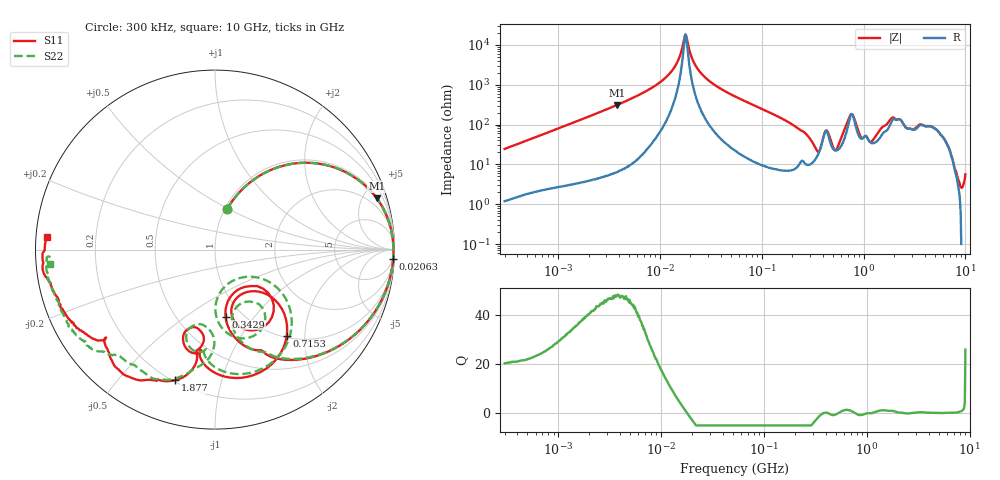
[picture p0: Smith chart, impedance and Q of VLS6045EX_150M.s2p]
! S-Parameter Data Generated by TDK Corporation
! Copyright(C) 2019 TDK Corporation.
! All Rights Reserved.
! TDK P/N: VLS6045EX-150M (Inductor)
! Property: L=15uH at 100kHz
! Size(LxWxT): 6x6x4.5mm
! Model Type: s2p (Touchstone File Format Version 1.0)
! Frequency: DC=Yes Start=0.3MHz Stop=10000MHz 802points Log-sweep
! Model Generated on May 10, 2019
! Port Assignments:
!  1 ---@@@--- 2
! Applicable Conditions:
!  Temperature = 25 degC
!  DC Bias Current = 0 A
!  Small Signal Operation
! Terms and conditions regarding TDK Simulation Models
! (1)This simulation model is being provided solely for informational purposes. Please refer to the specifications of the products in terms of detailed characteristics of such products.
! (2)In no event shall TDK Corporation of any of its subsidiaries be liable for any loss or damage arising, directly or indirectly,
!  From any information contained in this simulation model, including, but not limited to loss or damages arising from any inaccuracies, omissions or errors in connection with such information.
! (3)Any and all copyrights on this simulation model are owned by TDK Corporation.
!  Duplication or redistribution of this simulation model without prior written permission from TDK Corporation is prohibited.
! (4)This simulation model is subject to any modification or change without any prior notice.
! (5)Neither TDK Corporation nor any of its subsidiaries shall make any warranty, express or implied,
!  Including but not limited to the correctness, implied warranties of merchantability and fitness for a particular purpose with respect to this simulation models.
! (6)The use of this simulation model shall be deemed to have consented to the terms and conditions hereof.
# Hz S MA R 50
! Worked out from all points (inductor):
!   801 points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, 300 kHz to 10 GHz, reference 50 ohm
!   read as one part in series: L = 12.9 uH near 318.3 kHz
!   highest Q = 48 at 3.777 MHz (marker M1), where L = 12.9 uH
!   self-resonance near 17.86 MHz
!   S11 on the Smith chart (normalised r, x): 300 kHz: 1.03, +0.49; 20.63 MHz: 4, -38; 342.9 MHz: 0.84, -0.73; 715.3 MHz: 1.02, -1.63; 1.877 GHz: 0.21, -0.72; 10 GHz: 0.03, +0.04
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300000  0.2337 73.5  0.9607 -13.7  0.961 -13.7  0.2334 73.5
1713600  0.7936 35.8  0.5879 -52.7  0.588 -52.7  0.7937 35.8
3777497  0.945 17.6  0.3081 -71.2  0.3082 -71.2  0.945 17.6
9671944  0.9907 4.5  0.09293 -82.5  0.09296 -82.5  0.9909 4.5
1.405002e7  0.994 0.8  0.03512 -80.6  0.03513 -80.6  0.9942 0.8
1.786051e7  0.9944 -1.5  0.005483 -5.1  0.005482 -5.1  0.9946 -1.5
2.063197e7  0.9941 -3.0  0.02097 71.4  0.02097 71.4  0.9942 -2.9
2.856806e7  0.9914 -6.4  0.06883 78.5  0.06885 78.5  0.9916 -6.3
5.477226e7  0.9734 -15.7  0.1901 71.9  0.1901 71.9  0.9736 -15.6
1.69821e8  0.8005 -48.8  0.5598 38.7  0.5598 38.7  0.8018 -48.2
3.126428e8  0.4803 -78.5  0.7874 2.2  0.7874 2.2  0.4934 -75.9
3.428535e8  0.3778 -81.0  0.8039 -7.0  0.8038 -7.1  0.4055 -76.6
3.816958e8  0.2585 -62.1  0.7532 -20.8  0.7533 -20.8  0.3343 -61.6
4.568044e8  0.5079 -59.7  0.593 -12.9  0.593 -12.9  0.519 -72.5
5.911415e8  0.2904 -56.9  0.7494 -43.8  0.7494 -43.8  0.1998 -60.6
7.152593e8  0.6266 -50.4  0.3995 -70.0  0.3996 -70.0  0.5896 -43.5
9.445544e8  0.6121 -97.5  0.5105 -40.1  0.5104 -40.1  0.5987 -95.2
1.307877e9  0.4475 -105.2  0.5605 -80.0  0.5598 -80.1  0.4252 -102.6
1.767019e9  0.6812 -100.8  0.2683 -122.5  0.2675 -122.6  0.7274 -104.6
1.876852e9  0.7605 -107.0  0.1973 -123.8  0.1964 -123.8  0.7757 -110.7
2.568366e9  0.8394 -133.9  0.1587 -100.4  0.1589 -100.0  0.7958 -132.0
1e10  0.9382 175.6  0.04314 -155.2  0.04282 -155.0  0.9224 -175.1
